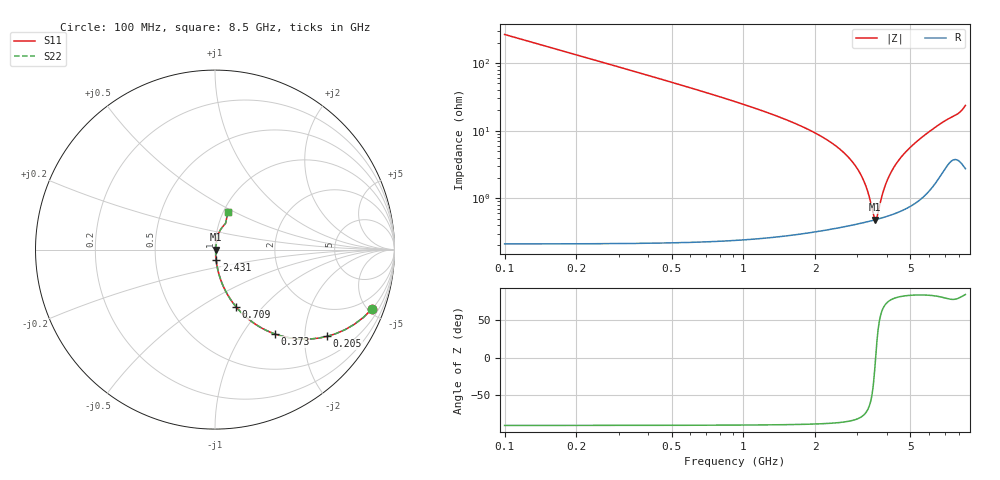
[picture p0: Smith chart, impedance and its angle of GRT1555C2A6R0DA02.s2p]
!Murata Part Number: GRT1555C2A6R0DA02
!These Parameters are Measured in Series Mode Connection
!Data Generated on Jun 19, 2026
!  o--ll--o
!Port1  Port2
!  o------o
!Operation Temp=25[degC], DC Bias Voltage=0[V]
!Freq. Start=100[MHz] Stop=9[GHz] 401[Steps]
# Hz S RI R 50
!Freq.(Hz) S11(Real) S11(Imag) S21(Real) S21(Imag) S12(Real) S12(Imag) S22(Real) S22(Imag)
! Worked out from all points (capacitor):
!   401 points, 100 MHz to 8.5 GHz, reference 50 ohm
!   read as one part in series: C = 6 pF near 142 MHz
!   lowest |Z| = 482 mohm at 3.565 GHz (marker M1)
!   series resonance near 3.578 GHz, so ESL is about 330 pH
!   S11 on the Smith chart (normalised r, x): 100 MHz: 1.00, -5.30; 205 MHz: 1.00, -2.58; 373 MHz: 1.00, -1.41; 709 MHz: 1.00, -0.72; 2.431 GHz: 1.01, -0.12; 8.5 GHz: 1.05, +0.47
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1e8  0.8752 -0.3301  0.1248 0.3301  0.1248 0.3301  0.8752 -0.3301
2.05e8  0.6244 -0.4835  0.3756 0.4835  0.3756 0.4835  0.6244 -0.4835
3.73e8  0.3316 -0.4693  0.6684 0.4693  0.6684 0.4693  0.3316 -0.4693
5.2e8  0.2008 -0.3984  0.7992 0.3984  0.7992 0.3984  0.2008 -0.3984
7.09e8  0.1161 -0.3173  0.8839 0.3173  0.8839 0.3173  0.1161 -0.3173
1.024e9  0.0558 -0.2245  0.9442 0.2245  0.9442 0.2245  0.0558 -0.2245
1.507e9  0.0233 -0.1417  0.9767 0.1417  0.9767 0.1417  0.0233 -0.1417
2.431e9  0.00706 -0.059  0.9929 0.059  0.9929 0.059  0.00706 -0.059
2.914e9  0.00501 -0.0311  0.995 0.0311  0.995 0.0311  0.00501 -0.0311
3.229e9  0.00462 -0.0156  0.9954 0.0156  0.9954 0.0156  0.00462 -0.0156
3.355e9  0.00461 -0.00979  0.9954 0.00979  0.9954 0.00979  0.00461 -0.00979
3.502e9  0.0047 -0.00327  0.9953 0.00327  0.9953 0.00327  0.0047 -0.00327
3.565e9  0.00477 -0.000542  0.9952 0.000542  0.9952 0.000542  0.00477 -0.000542
3.628e9  0.00486 0.00215  0.9951 -0.00215  0.9951 -0.00215  0.00486 0.00215
3.796e9  0.00516 0.00914  0.9948 -0.00914  0.9948 -0.00914  0.00516 0.00914
3.943e9  0.00551 0.0151  0.9945 -0.0151  0.9945 -0.0151  0.00551 0.0151
4.3e9  0.00671 0.029  0.9933 -0.029  0.9933 -0.029  0.00671 0.029
4.867e9  0.00967 0.0503  0.9903 -0.0503  0.9903 -0.0503  0.00967 0.0503
5.707e9  0.0173 0.0815  0.9827 -0.0815  0.9827 -0.0815  0.0173 0.0815
7.114e9  0.0472 0.1317  0.9528 -0.1317  0.9528 -0.1317  0.0472 0.1317
7.954e9  0.062 0.1603  0.938 -0.1603  0.938 -0.1603  0.062 0.1603
8.5e9  0.0748 0.2112  0.9252 -0.2112  0.9252 -0.2112  0.0748 0.2112
